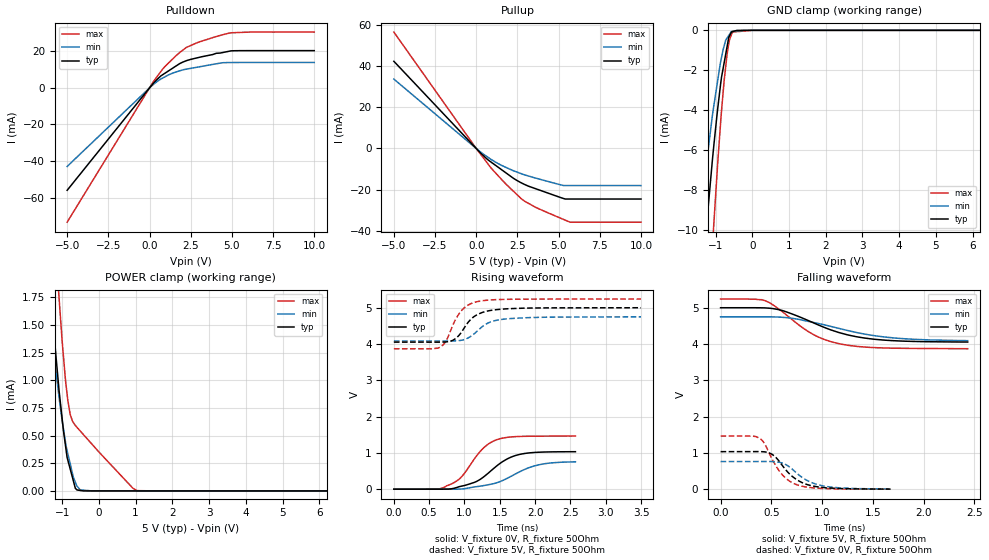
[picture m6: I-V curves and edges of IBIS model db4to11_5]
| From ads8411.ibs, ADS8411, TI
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|   db4to11_5 Model
[Model]   db4to11_5
Model_type   3-state
Polarity   Non-Inverting
Vmeas = 2.5
Vref = 2.5
Cref = 20pF
Rref = 50
|   typ   min   max
|   (nom PVT)   (fast PVT)   (slow PVT)
|C_comp from frequency sweep method (F=1MHz)
|C_comp   3.284e-12   3.239e-12   3.333e-12
|ON state : BUFFER OUTPUT TURNED HIGH
|C_comp   3.284e-12   3.239e-12   3.333e-12
|OFF state: BUFFER IN HIGH IMPEDANCE
|C_comp   3.270e-12   3.235e-12   3.307e-12
|C_comp from LC tank measurement(L=1nH)
|Resonant Frequency(Hz)   3.040e+09   3.060e+09   3.000e+09
C_comp   2.744e-12   2.708e-12   2.817e-12
|ON state : BUFFER OUTPUT TURNED HIGH
|Resonant Frequency(Hz)   3.050e+09   3.070e+09   3.010e+09
|C_comp   2.726e-12   2.690e-12   2.799e-12
|OFF state: BUFFER IN HIGH IMPEDANCE
|Resonant Frequency(Hz)   3.040e+09   3.060e+09   3.000e+09
|C_comp   2.744e-12   2.708e-12   2.817e-12
| Where nom  PVT is Nominal Process, 5V, 40C
|   Fast PVT is Strong Process,  5.25V, -40C
|   Slow PVT is Weak Process,   4.75V, 100C
[Voltage Range]   5   4.75   5.25
|Ambient Temperature   25   85   -40
|Junction Temperature
[Temperature Range]   40   100   -40
[Pullup Reference]   5   4.75   5.25
[Pulldown Reference]   0   0   0
[Power Clamp Reference]   5   4.75   5.25
[GND Clamp Reference]   0   0   0
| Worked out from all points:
|   slope of the pulldown table from 0 to 0.75 V, typ, clamps not added: 108 ohm
|   slope of the pullup table from 0 to 0.75 V, typ, clamps not added: 131 ohm
|   GND clamp passes 1 mA (typ) near -0.70 V on its own axis
|   POWER clamp passes 1 mA (typ) near -1.11 V on its own axis
|   falling waveform, V_fixture 5V, R_fixture 50Ohm: 20-80 % time 544ps typ, 656ps min, 431ps max; typ from 5 V to 4.05 V
|   rising waveform, V_fixture 0V, R_fixture 50Ohm: 20-80 % time 435ps typ, 520ps min, 355ps max; typ from 0 V to 1.03 V
|   rising waveform, V_fixture 5V, R_fixture 50Ohm: 20-80 % time 258ps typ, 288ps min, 225ps max; typ from 4.05 V to 5 V
|   falling waveform, V_fixture 0V, R_fixture 50Ohm: 20-80 % time 223ps typ, 241ps min, 197ps max; typ from 1.03 V to 0.002 V
[Pulldown]
|   Voltage   I(typ)   I(min)   I(max)
-5V       -56.07mA   -43.01mA   -73.51mA
252mV     2.669mA    2.026mA    3.652mA
700mV     6.638mA    4.914mA    9.138mA
924mV     7.959mA    6.012mA    11.61mA
1.825V    13.27mA    9.335mA    19.33mA
2.226V    14.86mA    10.26mA    22.11mA
2.94V     16.57mA    11.41mA    24.93mA
4.052V    18.96mA    13.2mA     28.12mA
4.403V    19.29mA    13.74mA    29.01mA
4.956V    20.3mA     13.89mA    30.18mA
10V       20.41mA    13.94mA    30.56mA
[GND Clamp]
|   Voltage   I(typ)   I(min)   I(max)
-5V       -1.352A    -1.001A    -1.995A
-1.533V   -18.82mA   -11.44mA   -26.71mA
-1.306V   -11.04mA   -7.542mA   -18.14mA
-1.176V   -8.353mA   -5.603mA   -13.75mA
-1.05V    -5.82mA    -3.813mA   -9.776mA
-865mV    -2.73mA    -1.605mA   -4.691mA
-766.5mV  -1.628mA   -781.2uA   -2.521mA
-687.7mV  -829.9uA   -389.3uA   -1.226mA
-640.5mV  -351.2uA   -257.7uA   -662.9uA
-570mV    -99.78uA   -61.37uA   -224uA
-84.44fV  0A         0A         0A
10V       0A         0A         0A
[Pullup]
|   Voltage   I(typ)   I(min)   I(max)
-5V       42.36mA    33.71mA    56.54mA
115.6fV   -8.124pA   -3.453pA   -3.426uA
475mV     -3.799mA   -2.975mA   -4.998mA
924mV     -6.747mA   -5.423mA   -9.72mA
1.596V    -10.65mA   -8.424mA   -15.56mA
2.27V     -14.56mA   -10.86mA   -20.86mA
2.767V    -16.82mA   -12.34mA   -24.63mA
3.602V    -19.53mA   -14.39mA   -28.57mA
5.18V     -24mA      -17.77mA   -34.06mA
5.405V    -24.56mA   -18mA      -34.83mA
5.696V    -24.56mA   -18mA      -35.81mA
10V       -24.56mA   -18.03mA   -35.81mA
[POWER Clamp]
|   Voltage   I(typ)   I(min)   I(max)
-5V       1.348A     997.9mA    1.981A
-1.517V   2.821mA    3.859mA    4.946mA
-1.31V    1.741mA    1.539mA    3.008mA
-1.085V   913.2uA    850.4uA    1.751mA
-997.5mV  646uA      630.8uA    1.345mA
-913.5mV  421.6uA    452.9uA    1.019mA
-845.2mV  278.9uA    336.7uA    818.2uA
-714mV    115.6uA    151.7uA    626.8uA
-595mV    8.714uA    43.23uA    574.2uA
-190mV    0A         0A         423.2uA
1.04V     0A         0A         2.581uA
10V       0A         0A         0A
[Ramp]
R_load = 50
|   typ   min   max
dV/dt_r   0.620252/4.34889e-10   0.456673/5.25186e-10   0.877789/3.54716e-10
dV/dt_f   0.568746/5.47114e-10   0.399296/6.71761e-10   0.822006/4.31834e-10
[Falling Waveform]
V_fixture = 5V
V_fixture_min = 4.75V
V_fixture_max = 5.25V
R_fixture = 50Ohm
|   Time   V(typ)   V(min)   V(max)
0s        5V         4.75V      5.239V
342ps     5V         4.75V      5.235V
442ps     4.995V     4.75V      5.189V
629ps     4.905V     4.732V     4.845V
800ps     4.723V     4.662V     4.464V
918ps     4.58V      4.593V     4.255V
1.17ns    4.313V     4.428V     4.007V
1.415ns   4.166V     4.276V     3.918V
1.696ns   4.093V     4.171V     3.886V
2.433ns   4.055V     4.093V     3.871V
[Rising Waveform]
V_fixture = 0V
V_fixture_min = 0V
V_fixture_max = 0V
R_fixture = 50Ohm
|   Time   V(typ)   V(min)   V(max)
0s        1.868nV    2.766nV    1.738nV
630ps     33.49uV    -25.39uV   3.849mV
814ps     10.54mV    234.5uV    141.7mV
964ps     85.73mV    5.418mV    351.9mV
1.186ns   228.1mV    73.13mV    953.6mV
1.338ns   443.6mV    121.7mV    1.245V
1.476ns   670.7mV    189.1mV    1.375V
1.824ns   974.5mV    519.9mV    1.455V
2.132ns   1.024V     700.4mV    1.462V
2.571ns   1.032V     754.1mV    1.463V
[Rising Waveform]
V_fixture = 5V
V_fixture_min = 4.75V
V_fixture_max = 5.25V
R_fixture = 50Ohm
|   Time   V(typ)   V(min)   V(max)
0s        4.052V     4.084V     3.869V
659ps     4.052V     4.084V     3.916V
746ps     4.06V      4.083V     4.11V
830ps     4.098V     4.085V     4.498V
949ps     4.304V     4.101V     4.901V
1.091ns   4.683V     4.214V     5.113V
1.193ns   4.823V     4.381V     5.173V
1.366ns   4.924V     4.606V     5.215V
1.628ns   4.973V     4.699V     5.233V
3.499ns   5V         4.75V      5.239V
[Falling Waveform]
V_fixture = 0V
V_fixture_min = 0V
V_fixture_max = 0V
R_fixture = 50Ohm
|   Time   V(typ)   V(min)   V(max)
0s        1.034V     761.5mV    1.463V
378ps     1.036V     762.5mV    1.409V
435ps     1.028V     763.4mV    1.243V
506ps     960.9mV    761.6mV    836.1mV
604ps     668.6mV    722mV      410.3mV
692ps     386.1mV    583.6mV    198.6mV
771ps     226.5mV    391.5mV    103.9mV
886ps     101.6mV    194.1mV    43.53mV
1.065ns   33.94mV    65.45mV    13.07mV
1.673ns   2.144mV    5.134mV    544.1uV
